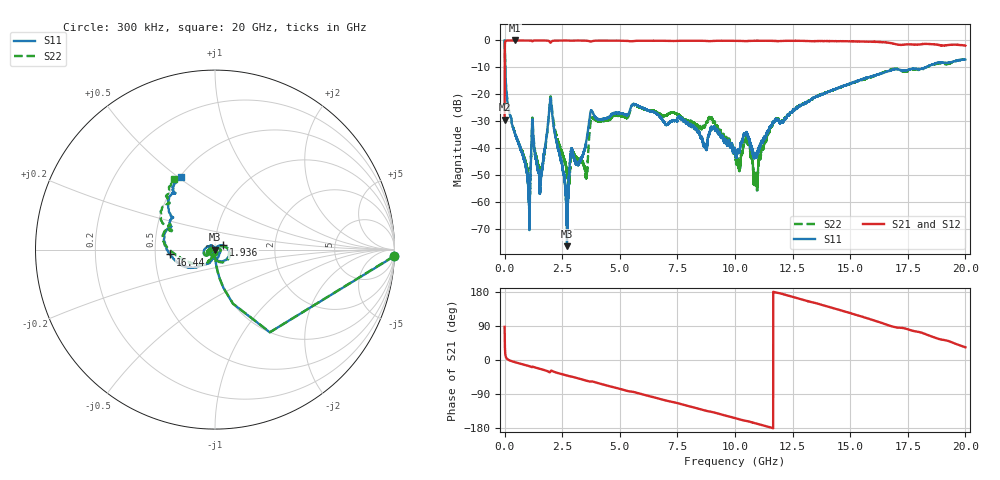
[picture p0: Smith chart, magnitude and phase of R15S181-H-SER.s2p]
!{R15S181}
!Johanson Technology Inc.
!www.johansontechnology.com
!Test Board Conditions:
!Substrate Type  RO4350B
!Substrate Thickness  20 mil
!Substrate Dk  3.66
!TL Type: GCPW
!TL Trace Width  34 mil
!TL Gap  10 mil
!Electrode orientation  Horizontal
!DUT TOPOLOGY	SERIES
!Mounting Pad LxW  26x52 mil
! Created Sat Feb  6 14:18:01 2021
# hz S ma R 50
! 2 Port Network Data from SP1.SP block
! freq  magS11  angS11  magS21  angS21  magS12  angS12  magS22  angS22
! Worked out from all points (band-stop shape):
!   20001 points, 300 kHz to 20 GHz, reference 50 ohm
!   highest |S21| = -0.01 dB at 462.3 MHz (marker M1); lowest = -29.4 dB at 300 kHz (marker M2)
!   |S21| within 3 dB of the highest: 8.891 MHz to end of sweep
!   lowest |S11| = -76.2 dB at 2.707 GHz (marker M3), VSWR 1.00, Z = 50 - j0.0142 ohm
!   |S11| at or under -10 dB: 26.46 MHz to 18.28 GHz (18.25 GHz wide, 199 % of centre); 18.27968 GHz to 18.28071 GHz (1.028 MHz wide, 0.00563 % of centre)
!   |S22| runs from -55.9 to 0.0 dB; largest |S21 - S12| = 0.017
!   S11 on the Smith chart (normalised r, x): 300 kHz: 3, -52; 1.936 GHz: 1.09, +0.05; 16.44 GHz: 0.60, -0.03; 20 GHz: 0.51, +0.51
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300000  0.9978 -2.2  0.03396 87.3  0.03417 87.8  0.9967 -2.1
1.053e8  0.08502 -85.8  0.9946 3.1  0.994 3.1  0.08529 -85.8
4.623e8  0.01811 -90.6  0.9987 -6.0  0.9972 -6.0  0.01858 -90.9
1.0363e9  0.001484 -90.0  0.9975 -15.7  0.9969 -15.6  0.003008 -68.1
1.2433e9  0.01755 -89.0  0.9908 -18.0  0.9911 -18.0  0.01899 -84.4
1.5913e9  0.003384 103.8  0.996 -24.3  0.9951 -24.3  0.003562 -24.4
1.9363e9  0.05022 28.0  0.9672 -31.8  0.9674 -31.8  0.05124 20.0
2.7073e9  0.0001553 -113.8  0.9945 -41.0  0.9946 -41.0  0.00329 -126.4
2.9093e9  0.01017 -64.9  0.9868 -43.9  0.9875 -43.9  0.009249 -90.7
3.3343e9  0.006433 -65.4  0.9934 -50.8  0.9931 -50.8  0.00586 158.7
3.5423e9  0.01308 -41.7  0.9867 -54.5  0.9883 -54.4  0.003018 77.9
3.7863e9  0.04919 -95.3  0.9644 -56.5  0.964 -56.5  0.03755 -115.0
6.6673e9  0.04205 154.6  0.9878 -101.4  0.9876 -101.4  0.04486 -161.2
8.9393e9  0.02323 156.2  0.972 -136.3  0.9731 -136.4  0.03592 -168.8
1.00003e10  0.009365 172.1  0.9844 -153.3  0.9851 -153.3  0.008309 142.9
1.05403e10  0.01744 -175.5  0.9729 -161.4  0.9739 -161.5  0.01359 168.4
1.08973e10  0.007381 -130.4  0.9831 -167.3  0.9842 -167.2  0.002689 -157.4
1.17123e10  0.03179 -102.3  0.978 179.1  0.978 179.1  0.03139 -109.7
1.33343e10  0.08231 -113.0  0.9681 152.8  0.967 152.7  0.0807 -118.5
1.64363e10  0.2506 -173.8  0.9296 96.3  0.9187 96.5  0.2564 -179.8
1.66673e10  0.2699 177.7  0.9063 91.5  0.8927 91.6  0.2818 174.2
2e10  0.4449 114.7  0.8016 33.5  0.793 33.4  0.4526 119.7
